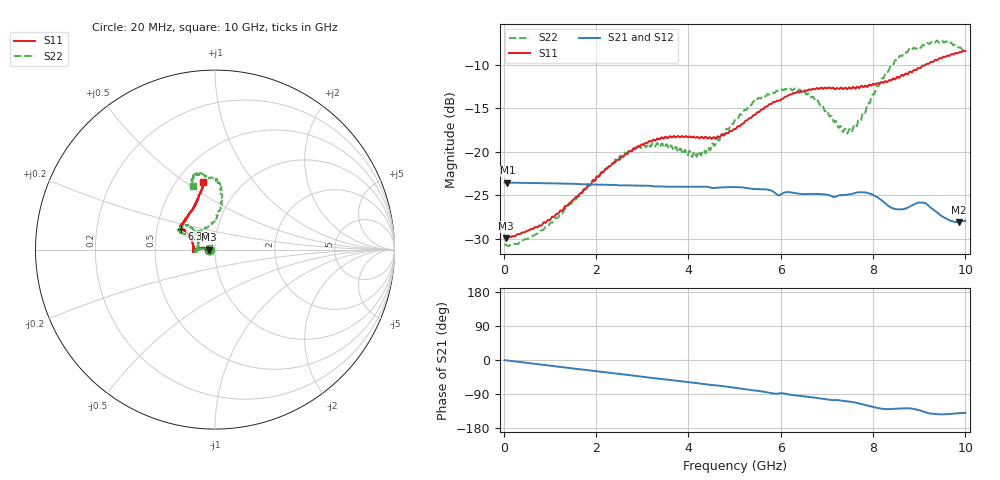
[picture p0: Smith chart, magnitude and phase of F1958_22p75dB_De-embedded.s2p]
! Integrated Device Technology
! Corporate Headquarters
! 6024 Silver Creek Valley Road
! San Jose, CA 95138  USA
! Phone:  1-408-284-8200
! Toll Free:  1-800-223-1366
! Webpage:  http://www.idt.com/
! Timing and RF Division
! 515 Groton Road, Suite 102
! Westford, MA 01886-6024
! Device:  F1958
! Description: 7-bit 0.25 dB Digital Step Attenuator
! Frequency:  0.001 -  6.000 GHz
! Package:  4x4 mm Thin QFN Plastic Package: 24 pin
! Ports:  2 RF, 12 DC
!  Pin  1  = D0
!  Pin  2  = VDD
!  Pin  3  = VMODE
!  Pin  4  = GND
!  Pin  5  = RF1  =  Port 1
!  Pin  6  = GND
!  Pin  7  = GND
!  Pin  8  = GND
!  Pin  9  = GND
!  Pin 10  = GND
!  Pin 11  = GND
!  Pin 12  = GND
!  Pin 13  = GND
!  Pin 14  = RF2  =  Port 2
!  Pin 15  = GND
!  Pin 16  = LE
!  Pin 17  = CLK
!  Pin 18  = DATA
!  Pin 19  = D6
!  Pin 20  = D5
!  Pin 21  = D4
!  Pin 22  = D3
!  Pin 23  = D2
!  Pin 24  = D1
! State:  91
! Atten State:  22.75 dB
! Voltage:  +3.30 Volts
! Current:  0.259 mA
! Data:  The device was measured on a F1958 evaluation board which has
!  individual transmission lines to the RF pins.  Data was collected
!  using a calibrated network analyzer.  The evaluation board was
!  de-embedded using Automatic Fixture Removal (AFR).
!  The reference plane is the edge of the package pin.
! Misc:
!  Action Tracker AT0419
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# GHz S dB R 50
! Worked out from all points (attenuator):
!   500 points, 20 MHz to 10 GHz, reference 50 ohm
!   highest |S21| = -23.55 dB at 80 MHz (marker M1); lowest = -28.1 dB at 9.86 GHz (marker M2)
!   lowest |S11| = -30.0 dB at 40 MHz (marker M3), VSWR 1.07, Z = 46.9 - j0.0426 ohm
!   |S11| at or under -10 dB: start of sweep to 9.132 GHz
!   |S22| runs from -30.9 to -7.2 dB; largest |S21 - S12| = 0.00033
!   S11 on the Smith chart (normalised r, x): 20 MHz: 0.94, -0.00; 6.36 GHz: 0.67, +0.16; 10 GHz: 0.67, +0.59
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0.02  -29.93 -178.9  -23.55 -0.3  -23.55 -0.3  -30.73 -178.8
0.04  -29.95 -179.2  -23.55 -0.6  -23.55 -0.6  -30.69 -178.2
0.08  -29.87 179.4  -23.55 -1.2  -23.55 -1.2  -30.84 -178.4
0.84  -28.36 171.1  -23.62 -12.5  -23.61 -12.5  -29.05 176.5
1.7  -24.73 171.0  -23.75 -25.1  -23.74 -25.0  -24.62 175.0
2.62  -20.33 177.0  -23.87 -38.4  -23.85 -38.4  -20.09 -179.0
3.36  -18.55 -175.8  -24.00 -49.4  -24.00 -49.5  -19.31 -172.1
4.24  -18.45 -179.2  -24.03 -61.9  -24.05 -62.0  -20.01 166.0
4.64  -18.21 171.6  -24.14 -67.4  -24.15 -67.4  -18.52 148.1
5.02  -17.38 160.7  -24.07 -73.6  -24.08 -73.6  -16.23 137.8
5.58  -15.13 150.5  -24.33 -82.7  -24.34 -82.7  -13.78 138.3
6.36  -13.12 148.0  -24.80 -94.0  -24.82 -94.0  -13.03 151.6
6.68  -12.79 146.6  -24.86 -98.3  -24.88 -98.2  -13.71 152.7
7.3  -12.60 140.8  -25.01 -107.0  -25.01 -106.9  -17.04 131.8
7.5  -12.62 138.1  -24.92 -110.0  -24.92 -109.9  -17.38 113.7
7.9  -12.39 128.9  -24.77 -121.0  -24.77 -121.0  -14.39 87.7
8.34  -11.77 118.9  -26.26 -129.8  -26.25 -129.9  -10.63 82.2
8.68  -11.13 112.2  -26.58 -127.7  -26.58 -127.4  -8.50 86.8
9.02  -10.37 107.7  -25.86 -133.2  -25.86 -133.3  -8.03 94.8
9.26  -9.62 104.7  -26.49 -141.5  -26.51 -141.7  -7.37 99.5
9.86  -8.55 99.8  -28.12 -140.3  -28.13 -140.1  -7.99 108.2
10  -8.41 99.7  -27.94 -139.4  -27.97 -139.3  -8.48 108.8
